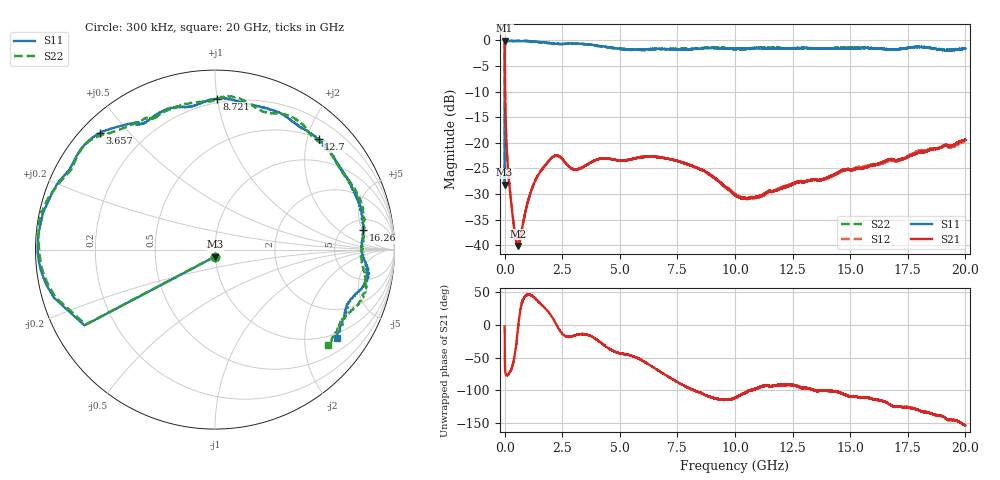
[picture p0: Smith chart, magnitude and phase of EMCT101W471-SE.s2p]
!EMCT101W471
!Johanson Technology Inc.
!www.johansontechnology.com
!Test Board Conditions:
!Substrate Type  RO4350B
!Substrate Thickness  10 mil
!Substrate Dk  3.66
!TL Type: GCPW
!TL Trace Width  22 mil
!TL Gap  14 mil
!PART MODE SINGLE ENDED (AKA BYPASS)
!DUT TOPOLOGY	SERIES-SHUNT
# MHz S  dB  R 50
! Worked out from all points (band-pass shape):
!   20001 points, 300 kHz to 20 GHz, reference 50 ohm
!   highest |S21| = -0.03 dB at 300 kHz (marker M1); lowest = -40.2 dB at 576.3 MHz (marker M2)
!   |S21| within 3 dB of the highest: start of sweep to 7.598 MHz
!   lowest |S11| = -28.2 dB at 300 kHz (marker M3), VSWR 1.08, Z = 49.8 - j3.9 ohm
!   |S11| at or under -10 dB: start of sweep to 2.658 MHz
!   |S22| runs from -28.3 to -0.1 dB; largest |S21 - S12| = 0.006
!   S11 on the Smith chart (normalised r, x): 300 kHz: 1.00, -0.08; 3.657 GHz: 0.05, +0.42; 8.721 GHz: 0.17, +1.00; 12.7 GHz: 0.51, +2.21; 16.26 GHz: 7.25, +5.11; 20 GHz: 0.87, -2.86
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0.3  -28.16 -90.3  -0.03 -2.3  -0.01 -2.3  -28.29 -90.8
105.298  -0.14 -176.6  -22.20 -76.9  -22.16 -77.0  -0.22 -176.6
175.297  -0.12 -179.1  -26.79 -74.8  -26.74 -74.8  -0.17 -179.0
311.295  -0.10 178.4  -32.74 -65.6  -32.67 -65.9  -0.15 178.1
467.293  -0.11 176.3  -38.29 -40.1  -38.21 -39.9  -0.11 175.6
576.291  -0.12 174.9  -40.16 -6.7  -40.06 -7.0  -0.09 174.0
1203.282  -0.24 166.0  -28.74 44.1  -28.76 44.3  -0.18 165.0
1879.272  -0.46 156.9  -23.77 20.8  -23.70 20.7  -0.56 155.7
2286.266  -0.67 151.5  -22.48 -1.8  -22.44 -2.1  -0.74 151.2
3334.25  -0.67 138.1  -24.88 -14.1  -24.89 -13.9  -0.67 139.2
3657.245  -0.80 134.5  -24.05 -15.8  -24.04 -15.8  -0.83 136.3
5100.224  -1.75 121.5  -23.44 -44.0  -23.48 -43.9  -1.64 117.9
6667.2  -1.65 108.6  -22.83 -69.4  -22.76 -69.7  -1.74 110.4
8721.169  -1.50 89.3  -25.64 -107.2  -25.71 -107.4  -1.39 87.7
10000.15  -1.60 75.0  -30.13 -111.4  -30.04 -110.9  -1.70 73.3
10962.14  -1.49 64.2  -30.57 -96.6  -30.66 -97.2  -1.49 63.5
12704.11  -1.46 46.9  -27.73 -93.3  -27.67 -93.6  -1.58 45.4
13334.1  -1.53 38.7  -27.25 -98.6  -27.20 -98.4  -1.57 36.6
16264.06  -1.60 7.5  -24.04 -114.8  -24.16 -116.7  -1.65 3.9
16667.05  -1.75 2.5  -23.23 -120.3  -23.48 -120.1  -1.76 -0.6
17909.03  -1.32 -10.2  -22.04 -128.9  -21.79 -128.8  -1.32 -15.4
20000  -1.53 -35.9  -19.42 -153.2  -19.64 -150.7  -1.69 -40.1
